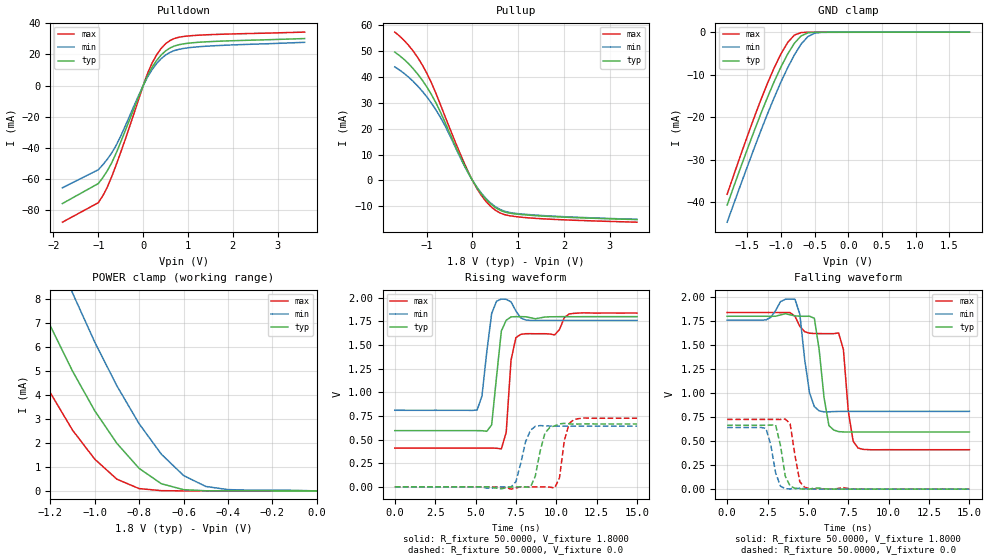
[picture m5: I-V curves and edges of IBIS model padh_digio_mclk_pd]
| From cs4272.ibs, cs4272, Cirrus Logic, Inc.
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|   Model mclkp
[Model]  padh_digio_mclk_pd
Model_type I/O
Polarity   Non-Inverting
Enable   Active-High
Vinl =   0.6250V
Vinh =   0.9750V
C_comp   5.0000pF   5.0000pF   5.0000pF
[Temperature Range]   25.0000   85.0000   -40.0000
[Voltage Range]   1.8000V   1.6200V   1.9800V
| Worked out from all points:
|   slope of the pulldown table from 0 to 0.27 V, typ, clamps not added: 18.2 ohm
|   slope of the pullup table from 0 to 0.27 V, typ, clamps not added: 39.9 ohm
|   GND clamp passes 1 mA (typ) near -0.71 V on its own axis
|   POWER clamp passes 1 mA (typ) near -0.81 V on its own axis
|   rising waveform, R_fixture 50.0000, V_fixture 1.8000: 20-80 % time 438ps typ, 379ps min, 521ps max; typ from 0.595 V to 1.8 V
|   rising waveform, R_fixture 50.0000, V_fixture 0.0: 20-80 % time 520ps typ, 576ps min, 413ps max; typ from 0 V to 0.665 V
|   falling waveform, R_fixture 50.0000, V_fixture 1.8000: 20-80 % time 520ps typ, 448ps min, 587ps max; typ from 1.8 V to 0.595 V
|   falling waveform, R_fixture 50.0000, V_fixture 0.0: 20-80 % time 410ps typ, 480ps min, 433ps max; typ from 0.666 V to 0 V
[Pulldown]
|Voltage   I(typ)   I(min)   I(max)
-1.8V     -75.65mA   -65.54mA   -87.6mA
-1V       -62.83mA   -53.94mA   -75.11mA
-900mV    -59.08mA   -50.81mA   -70.72mA
-800mV    -54.69mA   -47.26mA   -65.17mA
-600mV    -43.2mA    -38.24mA   -50.73mA
-100mV    -7.132mA   -6.253mA   -8.793mA
100mV     6.434mA    5.61mA     7.989mA
300mV     16.15mA    14.17mA    19.75mA
500mV     22.27mA    19.64mA    26.88mA
700mV     25.47mA    22.55mA    30.3mA
1.1V      27.52mA    24.61mA    32.13mA
3.6V      30.22mA    27.8mA     34.37mA
[Pullup]
|Voltage   I(typ)   I(min)   I(max)
-1.7V     49.68mA    43.95mA    57.42mA
-1.4V     45.22mA    40.02mA    52.35mA
-1.1V     38.85mA    34.57mA    44.78mA
-900mV    33.31mA    29.97mA    37.86mA
-700mV    26.44mA    24.4mA     29.28mA
-300mV    10.43mA    10.01mA    11.63mA
0V        0A         0A         0A
200mV     -5.304mA   -5.08mA    -5.942mA
500mV     -10.49mA   -10.16mA   -11.53mA
700mV     -12.2mA    -11.93mA   -13.23mA
1.1V      -13.26mA   -13.04mA   -14.3mA
3.6V      -15.16mA   -15.06mA   -16.17mA
[GND_clamp]
|Voltage   I(typ)   I(min)   I(max)
-1.8V     -40.65mA   -44.66mA   -38.1mA
-1.5V     -27.51mA   -31.59mA   -24.46mA
-1.3V     -19.2mA    -23.2mA    -15.94mA
-1.1V     -11.57mA   -15.34mA   -8.337mA
-1V       -8.149mA   -11.68mA   -5.09mA
-900mV    -5.124mA   -8.342mA   -2.406mA
-800mV    -2.578mA   -5.315mA   -667.9uA
-700mV    -856.8uA   -2.778mA   -82.45uA
-600mV    -148.6uA   -1.028mA   -7.033uA
-500mV    -14.64uA   -235.2uA   -2.45uA
-400mV    -2.251uA   -52.12uA   -1.809uA
1.8V      1.325uA    27.96uA    1.606uA
[POWER_clamp]
|Voltage   I(typ)   I(min)   I(max)
-1.8V     21.57mA    26.57mA    17.86mA
-1.4V     11.23mA    15.41mA    7.973mA
-1.3V     8.972mA    12.88mA    5.92mA
-1.2V     6.885mA    10.49mA    4.095mA
-1.1V     4.999mA    8.257mA    2.537mA
-1V       3.346mA    6.21mA     1.327mA
-900mV    1.983mA    4.379mA    488.8uA
-800mV    940.6uA    2.803mA    97.35uA
-700mV    300.3uA    1.534mA    11.09uA
-600mV    53.11uA    643.9uA    2.159uA
-400mV    1.652uA    54.56uA    1.609uA
0V        0A         0A         0A
[Ramp]
| variable   typ   min   max
dV/dt_r  0.3992/0.4672n   0.2953/0.6593n   0.5474/0.3941n
dV/dt_f  0.7231/0.4499n   0.5315/0.5846n   0.9226/0.3087n
R_load = 50.0000
[Rising Waveform]
R_fixture= 50.0000
V_fixture= 1.8000
V_fixture_min= 1.9800
V_fixture_max= 1.6200
|time   V(typ)   V(min)   V(max)
0s        594.8mV    810.1mV    410.3mV
5.1ns     594.7mV    813.9mV    410.3mV
5.4ns     594.1mV    961.3mV    410.3mV
5.7ns     587.6mV    1.431V     410.4mV
6ns       656.2mV    1.834V     410.4mV
6.6ns     1.649V     1.986V     401.7mV
6.9ns     1.762V     1.983V     576.1mV
7.2ns     1.798V     1.956V     1.341V
7.5ns     1.8V       1.861V     1.578V
15ns      1.8V       1.76V      1.838V
[Rising Waveform]
R_fixture= 50.0000
V_fixture= 0.0
|time   V(typ)   V(min)   V(max)
0s        0V         115.8uV    0V
7.2ns     -868.3uV   489.5uV    -24.18mV
7.5ns     -141.4uV   54.48mV    -10.98mV
8.4ns     -3.518mV   597.1mV    -122.9uV
9.3ns     569mV      645.7mV    158.6uV
9.9ns     645.1mV    642.5mV    -12.46mV
10.2ns    666.1mV    642mV      96.78mV
10.5ns    671.5mV    641.8mV    491.4mV
10.8ns    666.1mV    641.8mV    670.8mV
15ns      665.4mV    641.9mV    726.2mV
[Falling Waveform]
R_fixture= 50.0000
V_fixture= 1.8000
V_fixture_min= 1.9800
V_fixture_max= 1.6200
|time   V(typ)   V(min)   V(max)
0s        1.8V       1.76V      1.839V
4.2ns     1.804V     1.976V     1.8V
5.1ns     1.8V       1.004V     1.623V
5.4ns     1.779V     859mV      1.62V
6ns       952.7mV    804.8mV    1.619V
6.6ns     615.5mV    807.5mV    1.619V
7.2ns     595.7mV    809.6mV    1.453V
7.5ns     594.8mV    809.8mV    814.5mV
8.1ns     594.9mV    809.8mV    428.4mV
15ns      594.8mV    809.8mV    410.3mV
[Falling Waveform]
R_fixture= 50.0000
V_fixture= 0.0
|time   V(typ)   V(min)   V(max)
0s        665.5mV    641.6mV    726.2mV
2.4ns     665.3mV    632.9mV    726.2mV
2.7ns     666.6mV    463mV      726.2mV
3ns       668.2mV    170.7mV    726.1mV
3.3ns     457.1mV    30.68mV    725.7mV
3.6ns     134.2mV    5.373mV    729.1mV
3.9ns     31.98mV    1.155mV    681.7mV
4.5ns     2.43mV     9.563mV    76.47mV
4.8ns     533.3uV    6.573mV    19.71mV
15ns      -3.974uV   0V         885.9nV
